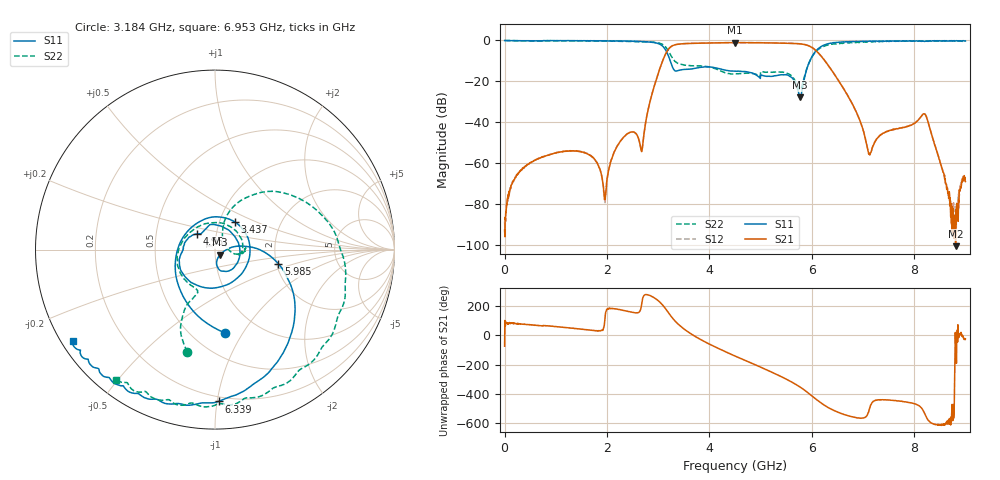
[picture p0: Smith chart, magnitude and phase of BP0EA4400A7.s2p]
!Agilent Technologies,E8358A,US40260310,A.06.04.32
!Agilent E8358A: A.06.04.32
!Date: Friday, November 22, 2019 00:20:16
!Correction: S11(Full 2 Port(1,2)) S21(Full 2 Port(1,2)) S12(Full 2 Port(1,2)) S22(Full 2 Port(1,2))
!S2P File: Measurements: S11, S21, S12, S22:
# Hz S  dB  R 50
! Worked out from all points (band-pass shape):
!   1601 points, 300 kHz to 9 GHz, reference 50 ohm
!   highest |S21| = -1.08 dB at 4.506 GHz (marker M1); lowest = -100.7 dB at 8.809 GHz (marker M2)
!   |S21| within 3 dB of the highest: 3.207 GHz to 6.04 GHz (2.833 GHz wide, 61.3 % of centre)
!   lowest |S11| = -27.9 dB at 5.771 GHz (marker M3), VSWR 1.08, Z = 52.8 - j3.05 ohm
!   |S11| at or under -10 dB: 3.234 GHz to 5.963 GHz (2.728 GHz wide, 59.3 % of centre)
!   |S22| runs from -24.1 to 0.0 dB; largest |S21 - S12| = 0.0098
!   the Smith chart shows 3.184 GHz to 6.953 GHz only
!   S11 on the Smith chart (normalised r, x): 3.184 GHz: 0.71, -0.84; 3.437 GHz: 1.19, +0.38; 4.95 GHz: 0.81, +0.14; 5.985 GHz: 2.05, -0.37; 6.339 GHz: 0.17, -1.01; 6.953 GHz: 0.03, -0.29
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300000  -0.07 -180.0  -92.88 -75.2  -88.72 -108.3  -0.01 -179.9
1.502125e9  -0.15 145.6  -54.63 40.0  -54.42 40.1  -0.24 114.9
1.96336e9  -0.23 129.0  -77.64 121.2  -79.12 128.4  -0.34 85.7
2.295224e9  -0.33 111.7  -48.29 170.3  -48.23 170.0  -0.46 56.1
2.683336e9  -0.58 76.8  -53.91 -135.6  -53.85 -135.2  -0.69 6.0
3.00395e9  -1.61 10.8  -15.90 -126.7  -15.83 -126.6  -1.23 -55.8
3.183944e9  -6.60 -83.1  -4.90 160.4  -4.86 160.4  -4.58 -105.1
3.43706e9  -14.42 53.9  -1.70 60.5  -1.67 60.3  -11.67 -112.1
4.022041e9  -13.03 -145.8  -1.26 -64.7  -1.20 -65.1  -13.10 -161.3
4.50015e9  -15.01 178.5  -1.08 -141.7  -1.03 -142.0  -16.37 78.3
4.505775e9  -15.03 178.2  -1.08 -142.7  -1.03 -142.8  -16.34 76.8
4.950135e9  -17.49 138.9  -1.10 150.4  -1.05 150.2  -17.18 -10.5
5.771358e9  -27.90 -45.7  -1.67 7.2  -1.63 7.1  -24.06 27.9
5.9851e9  -8.83 -12.6  -3.18 -48.1  -3.16 -48.0  -8.94 56.8
6.001975e9  -8.00 -16.9  -3.46 -52.9  -3.38 -52.9  -8.18 53.2
6.339464e9  -1.45 -88.7  -12.90 -135.1  -12.89 -135.8  -2.16 -28.9
6.952568e9  -0.51 -147.2  -40.10 155.2  -40.11 155.4  -0.81 -127.1
7.132562e9  -0.33 -156.4  -55.96 -133.3  -56.06 -134.5  -0.70 -144.3
7.5038e9  -0.28 -170.3  -44.19 -80.6  -44.18 -81.4  -0.50 -169.6
8.212526e9  -0.44 171.0  -36.19 -178.4  -36.12 -179.2  -0.34 167.3
8.808756e9  -0.22 160.4  -100.73 -53.3  -86.08 -106.1  -0.30 156.9
9e9  -0.26 157.5  -69.09 -26.9  -68.64 -25.7  -0.24 153.5
